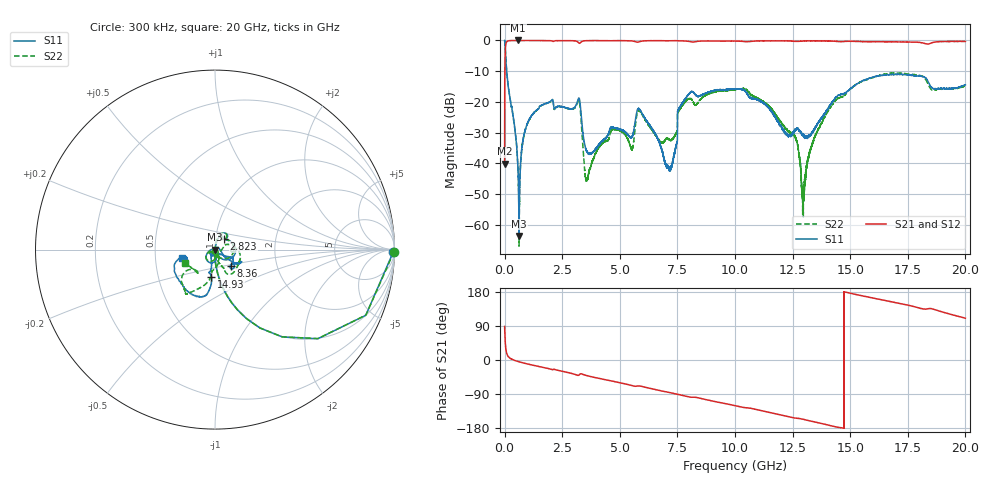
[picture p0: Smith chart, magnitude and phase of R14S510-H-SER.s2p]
!{R14S510}
!Johanson Technology Inc.
!www.johansontechnology.com
!Test Board Conditions:
!Substrate Type  RO4350B
!Substrate Thickness  20 mil
!Substrate Dk  3.66
!TL Type: GCPW
!TL Trace Width  36 mil
!TL Gap  12 mil
!Electrode orientation  Horizontal
!DUT TOPOLOGY	SERIES
!Mounting Pad LxW  26x36 mil
! Created Wed Nov 25 17:33:21 2020
! 2 Port Network Data from SP1.SP block
! freq  magS11  angS11  magS21  angS21  magS12  angS12  magS22  angS22
# khz S ma R 50
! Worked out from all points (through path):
!   20001 points, 300 kHz to 20 GHz, reference 50 ohm
!   highest |S21| = 0.00 dB at 594.3 MHz (marker M1); lowest = -40.2 dB at 300 kHz (marker M2)
!   group delay of S21, straight-line fit = 34.7 ps
!   lowest |S11| = -63.7 dB at 627.3 MHz (marker M3), VSWR 1.00, Z = 50.1 - j0.0349 ohm
!   |S11| at or under -10 dB: 90.04 MHz to end of sweep
!   |S22| runs from -67.0 to 0.0 dB; largest |S21 - S12| = 0.017
!   S11 on the Smith chart (normalised r, x): 300 kHz: open; 2.823 GHz: 1.10, +0.13; 8.36 GHz: 1.17, -0.21; 14.93 GHz: 0.92, -0.29; 20 GHz: 0.69, -0.07
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300  0.9936 -0.7  0.009821 88.6  0.00974 89.2  0.9971 -0.7
114300  0.2512 -76.2  0.967 13.7  0.9669 13.6  0.2524 -76.2
594300  0.005942 -89.2  0.9999 -4.2  0.999 -4.1  0.006268 -97.8
627300  0.0006552 -32.1  0.9992 -4.8  0.9997 -4.7  0.0005368 -135.1
1209300  0.06232 74.6  0.9966 -13.4  0.9962 -13.4  0.06178 77.8
2823300  0.07737 50.3  0.9923 -34.2  0.9921 -34.2  0.07641 56.8
3334300  0.05529 -57.0  0.9529 -36.6  0.9535 -36.6  0.04268 -65.9
3573300  0.01539 -55.6  0.9918 -41.3  0.991 -41.2  0.005636 -161.1
4697300  0.0387 -118.6  0.9907 -55.9  0.9911 -55.9  0.03585 -156.4
5519300  0.02675 -101.7  0.9815 -67.3  0.9815 -67.4  0.01669 -127.6
5833300  0.07764 -118.6  0.9504 -68.3  0.95 -68.3  0.07266 -124.7
6667300  0.02402 -175.2  0.9918 -79.7  0.9917 -79.7  0.02457 -139.3
7192300  0.008249 117.0  0.99 -86.2  0.9894 -86.2  0.02385 -91.2
7600300  0.08183 -35.7  0.9865 -91.8  0.9871 -91.8  0.07541 22.3
8360300  0.124 -45.6  0.9642 -99.2  0.964 -99.2  0.09464 3.1
1.00003e7  0.1625 -24.6  0.976 -120.4  0.9761 -120.5  0.1588 -41.5
1.25593e7  0.03238 -113.5  0.9695 -152.7  0.9693 -152.7  0.02924 -99.7
1.29643e7  0.02917 -163.6  0.9797 -156.6  0.9794 -156.6  0.001834 64.9
1.33343e7  0.03077 -134.7  0.9847 -161.9  0.9857 -161.9  0.01944 -34.7
1.49343e7  0.1542 -97.4  0.9694 177.3  0.97 177.0  0.1524 -98.4
1.66673e7  0.2743 -108.9  0.9534 155.3  0.9456 155.0  0.2906 -121.9
2e7  0.1901 -165.8  0.9621 110.3  0.9625 110.4  0.1837 -157.2
